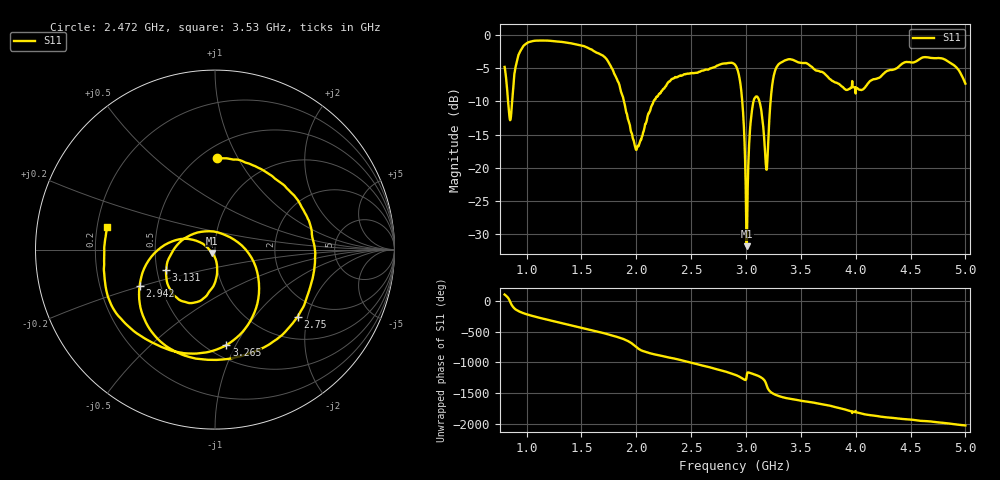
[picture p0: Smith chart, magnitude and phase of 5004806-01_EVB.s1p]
#  HZ  S  RI  R  50.00
! Rohde & Schwarz ZVA/B
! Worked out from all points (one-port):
!   1601 points, 800 MHz to 5 GHz, reference 50 ohm
!   lowest |S11| = -31.8 dB at 3.008 GHz (marker M1), VSWR 1.05, Z = 48.3 - j1.88 ohm
!   |S11| at or under -10 dB: 1.889 GHz to 2.158 GHz (269.2 MHz wide, 13.3 % of centre); 2.966 GHz to 3.069 GHz (102.9 MHz wide, 3.41 % of centre); 3.122 GHz to 3.224 GHz (101.9 MHz wide, 3.21 % of centre)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
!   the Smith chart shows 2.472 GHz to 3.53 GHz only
!   S11 on the Smith chart (normalised r, x): 2.472 GHz: 0.60, +0.83; 2.75 GHz: 1.51, -1.74; 2.942 GHz: 0.38, -0.20; 3.131 GHz: 0.56, -0.14; 3.265 GHz: 0.61, -0.92; 3.53 GHz: 0.24, +0.10
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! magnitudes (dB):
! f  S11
! 800 MHz  -4.8
! 849.9 MHz  -12.8
! 907.6 MHz  -4.4
! 970.6 MHz  -1.7
! 1.325 GHz  -1.1
! 1.703 GHz  -3.2
! 1.85 GHz  -7.8
! 2.005 GHz  -17.2
! 2.165 GHz  -9.8
! 2.375 GHz  -6.4
! 2.472 GHz  -5.8
! 2.75 GHz  -4.5
! 2.9 GHz  -4.5
! 2.942 GHz  -6.6
! 2.968 GHz  -10.4
! 2.992 GHz  -18.7
! 3.008 GHz  -31.8
! 3.063 GHz  -10.4
! 3.131 GHz  -10.6
! 3.186 GHz  -20.3
! 3.233 GHz  -8.4
! 3.265 GHz  -5.4
! 3.425 GHz  -3.7
! 3.53 GHz  -4.3
! 3.95 GHz  -8.0
! 4.475 GHz  -4.1
! 4.798 GHz  -3.6
! 5 GHz  -7.3
